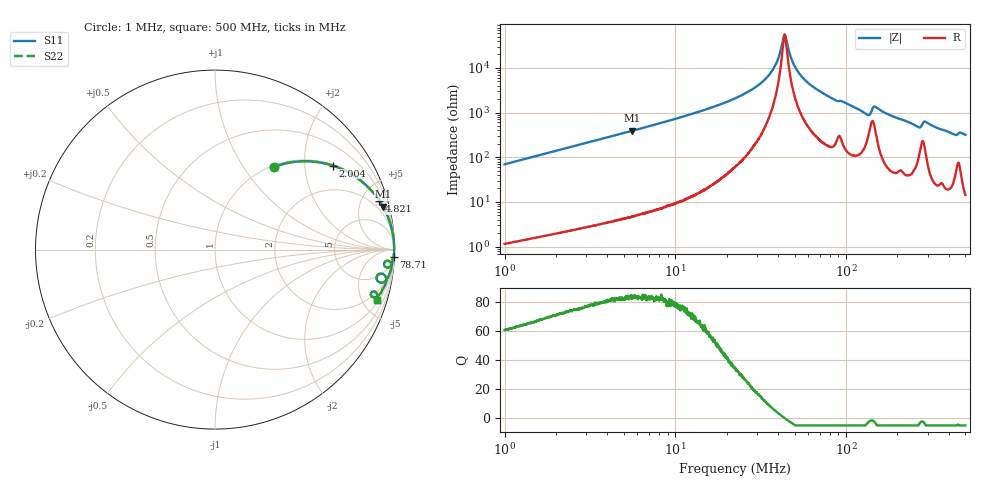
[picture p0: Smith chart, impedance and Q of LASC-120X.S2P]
!s-Parameter Generated by FASTRON Sdn. Bhd.
!FASTRON P/N : LASC-120X
!Keysight Technologies,E4991B,MY54100416,A.01.15
!Date: Mon Mar 16 09:49:28 2026
!Version  : Rev00 Mon Mar 16 09:49:28 2026
!Data & Calibration Information:
!PortZ  Port1:50+j0  Port2:50+j0
!When reading, reference impedance value at option line is always used.
!Remarks : This data is being provided solely for informational purposes.
!Freq	S11	S21	S12	S22
# Hz S dB R 50
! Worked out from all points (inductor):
!   1601 points, 1 MHz to 500 MHz, reference 50 ohm
!   read as one part in series: L = 11 uH near 1.032 MHz
!   highest Q = 83.7 at 5.61 MHz (marker M1), where L = 11.1 uH
!   self-resonance near 43.61 MHz
!   S11 on the Smith chart (normalised r, x): 1 MHz: 1.02, +1.39; 2.004 MHz: 1.04, +2.78; 4.821 MHz: 1.08, +6.71; 78.71 MHz: 5, -46; 500 MHz: 1.29, -6.36
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1000000  -4.93 54.5  -1.78 -34.5  -1.78 -34.5  -4.93 54.5
2004229  -1.87 35.5  -4.72 -53.7  -4.72 -53.7  -1.87 35.5
2820919  -1.06 27.0  -6.87 -62.3  -6.87 -62.3  -1.06 27.0
4821440  -0.40 16.5  -10.91 -72.8  -10.91 -72.8  -0.40 16.5
5610017  -0.30 14.3  -12.16 -75.0  -12.16 -75.0  -0.30 14.3
7957584  -0.15 10.0  -15.18 -79.3  -15.18 -79.3  -0.15 10.0
2.236068e7  -0.02 2.8  -26.35 -85.6  -26.35 -85.6  -0.02 2.8
2.923332e7  -0.02 1.6  -31.17 -85.4  -31.17 -85.4  -0.02 1.6
3.522469e7  -0.02 0.8  -36.69 -82.8  -36.69 -82.8  -0.02 0.8
3.927165e7  -0.01 0.4  -42.60 -76.6  -42.60 -76.6  -0.01 0.4
4.361384e7  -0.02 0.0  -54.92 -5.5  -54.92 -5.5  -0.02 0.0
4.464218e7  -0.02 -0.1  -52.84 38.1  -52.84 38.1  -0.02 -0.1
5.074715e7  -0.02 -0.6  -39.84 78.3  -39.84 78.3  -0.02 -0.6
6.307767e7  -0.02 -1.4  -31.94 83.2  -31.94 83.2  -0.02 -1.4
7.870937e7  -0.04 -2.5  -27.34 83.2  -27.34 83.2  -0.04 -2.5
1.32454e8  -0.29 -5.9  -19.42 69.4  -19.42 69.4  -0.29 -5.9
1.476717e8  -0.22 -3.9  -22.89 67.6  -22.89 67.6  -0.22 -3.9
1.77937e8  -0.11 -6.3  -19.19 80.2  -19.19 80.2  -0.11 -6.3
2.623928e8  -0.46 -11.2  -14.13 69.4  -14.13 69.4  -0.46 -11.2
2.91405e8  -0.39 -8.6  -16.32 69.1  -16.32 69.1  -0.39 -8.6
4.247389e8  -0.57 -16.4  -10.98 69.0  -10.98 69.0  -0.57 -16.4
5e8  -0.52 -17.2  -10.58 70.2  -10.58 70.2  -0.52 -17.2
